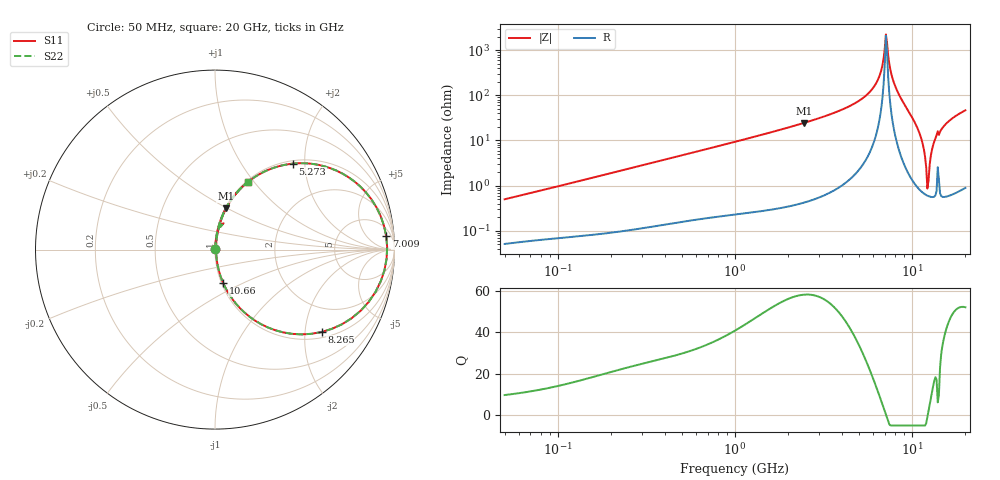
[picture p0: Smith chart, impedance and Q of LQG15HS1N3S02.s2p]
!Murata Part Number: LQG15HS1N3S02
!These Parameters are Measured in Series Mode Connection
!  o--[Z]--o
!Port1  Port2
!  o-------o
!Freq. Start=50[MHz] Stop=20[GHz], 401[Steps]
# Hz S RI R 50
!Freq.(Hz) S11(Real) S11(Imag) S21(Real) S21(Imag) S12(Real) S12(Imag) S22(Real) S22(Imag)
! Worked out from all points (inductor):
!   401 points, 50 MHz to 20 GHz, reference 50 ohm
!   read as one part in series: L = 1.56 nH near 51.52 MHz
!   highest Q = 58.2 at 2.456 GHz (marker M1), where L = 1.59 nH
!   self-resonance near 7.115 GHz
!   S11 on the Smith chart (normalised r, x): 50 MHz: 1.00, +0.01; 5.273 GHz: 1.06, +1.74; 7.009 GHz: 11, +19; 8.265 GHz: 1.16, -2.44; 10.66 GHz: 1.02, -0.39; 20 GHz: 1.02, +0.93
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5e7  0.000536 0.00495  0.9995 -0.00495  0.9995 -0.00495  0.000536 0.00495
1.364002e8  0.000938 0.013  0.9991 -0.013  0.9991 -0.013  0.000938 0.013
3.721004e8  0.00252 0.0348  0.9975 -0.0348  0.9975 -0.0348  0.00252 0.0348
1e9  0.0109 0.0922  0.9891 -0.0922  0.9891 -0.0922  0.0109 0.0922
2.456456e9  0.0603 0.2296  0.9397 -0.2296  0.9397 -0.2296  0.0603 0.2296
2.728004e9  0.0758 0.2562  0.9242 -0.2562  0.9242 -0.2562  0.0758 0.2562
5.273168e9  0.4328 0.4789  0.5672 -0.4789  0.5672 -0.4789  0.4328 0.4789
6.406762e9  0.8085 0.3524  0.1915 -0.3524  0.1915 -0.3524  0.8085 0.3524
6.701223e9  0.8989 0.2366  0.1011 -0.2366  0.1011 -0.2366  0.8989 0.2366
7.009217e9  0.954 0.0753  0.046 -0.0753  0.046 -0.0753  0.954 0.0753
7.222371e9  0.9561 -0.05  0.0439 0.05  0.0439 0.05  0.9561 -0.05
7.442007e9  0.9234 -0.1771  0.0766 0.1771  0.0766 0.1771  0.9234 -0.1771
7.784049e9  0.8112 -0.341  0.1888 0.341  0.1888 0.341  0.8112 -0.341
8.264682e9  0.5934 -0.4593  0.4066 0.4593  0.4066 0.4593  0.5934 -0.4593
9.316812e9  0.2222 -0.395  0.7778 0.395  0.7778 0.395  0.2222 -0.395
1.066139e10  0.0458 -0.1865  0.9542 0.1865  0.9542 0.1865  0.0458 -0.1865
1.149051e10  0.0136 -0.0809  0.9864 0.0809  0.9864 0.0809  0.0136 -0.0809
1.201863e10  0.00673 -0.0241  0.9933 0.0241  0.9933 0.0241  0.00673 -0.0241
1.238412e10  0.00594 0.0113  0.9941 -0.0113  0.9941 -0.0113  0.00594 0.0113
1.314879e10  0.0116 0.0772  0.9884 -0.0772  0.9884 -0.0772  0.0116 0.0772
1.396067e10  0.0476 0.1469  0.9524 -0.1469  0.9524 -0.1469  0.0476 0.1469
2e10  0.1829 0.3771  0.8171 -0.3771  0.8171 -0.3771  0.1829 0.3771
